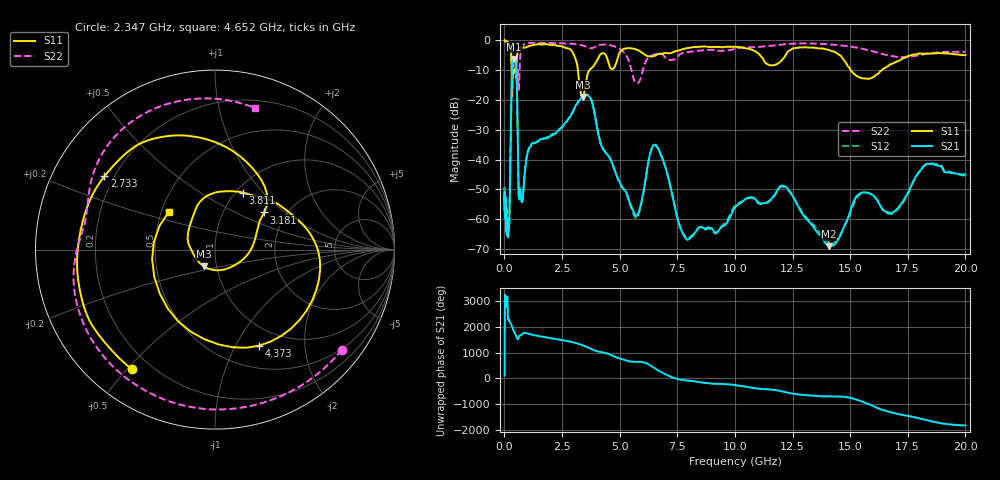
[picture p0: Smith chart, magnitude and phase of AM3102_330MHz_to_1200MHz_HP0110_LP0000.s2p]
! Date/Time: Tue, Sep 11, 2018 5:14 PM
! Network Analyzer: Agilent Technologies E8362B Rev: A.07.50.63
! Sweep from 0.010 to 20.000 GHz, 1601 Points, Sweep Type: LOG
! Power Supply: 4.949 V, 0.001 A
# Hz S DB R 50
!freq MagS11 AngS11 MagS21 AngS21 MagS12 AngS12 MagS22 AngS22
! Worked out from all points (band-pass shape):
!   1601 points, 10 MHz to 20 GHz, reference 50 ohm
!   highest |S21| = -6.20 dB at 420.4 MHz (marker M1); lowest = -69.0 dB at 14.07 GHz (marker M2)
!   |S21| within 3 dB of the highest: 339.9 MHz to 516.9 MHz (177 MHz wide, 41.3 % of centre)
!   lowest |S11| = -19.0 dB at 3.4 GHz (marker M3), VSWR 1.25, Z = 43.4 - j8.18 ohm
!   |S11| at or under -10 dB: 315.1 MHz to 377.6 MHz (62.48 MHz wide, 18 % of centre); 3.19 GHz to 3.687 GHz (496.7 MHz wide, 14.4 % of centre); 15.03 GHz to 16.37 GHz (1.34 GHz wide, 8.54 % of centre)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
!   |S22| runs from -16.5 to -0.2 dB; largest |S21 - S12| = 0.0059
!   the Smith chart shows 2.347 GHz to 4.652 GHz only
!   S11 on the Smith chart (normalised r, x): 2.347 GHz: 0.13, -0.52; 2.733 GHz: 0.16, +0.29; 3.181 GHz: 1.55, +0.73; 3.811 GHz: 1.07, +0.78; 4.373 GHz: 0.76, -1.25; 4.652 GHz: 0.55, +0.26
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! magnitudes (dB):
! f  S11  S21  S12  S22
! 10 MHz  0.0  -53.3  -50.3  -0.2
! 35.55 MHz  0.0  -58.5  -56.7  -0.3
! 126.4 MHz  -0.4  -65.4  -63.1  -0.7
! 217.2 MHz  -1.4  -58.5  -59.9  -1.5
! 420.4 MHz  -10.9  -6.2  -6.2  -7.1
! 447.2 MHz  -10.1  -6.3  -6.4  -7.2
! 530.6 MHz  -7.5  -11.7  -11.7  -12.5
! 635.6 MHz  -2.4  -53.2  -53.5  -15.9
! 1.59 GHz  -1.4  -33.1  -33.1  -0.8
! 2.347 GHz  -1.8  -30.0  -30.4  -0.9
! 2.733 GHz  -2.6  -26.8  -27.0  -1.0
! 3.181 GHz  -9.3  -20.7  -20.9  -1.3
! 3.4 GHz  -19.0  -18.7  -18.9  -1.7
! 3.811 GHz  -9.0  -20.9  -20.8  -2.6
! 4.373 GHz  -4.6  -37.4  -37.4  -1.4
! 4.652 GHz  -9.6  -40.7  -40.7  -1.7
! 5.652 GHz  -2.9  -58.3  -59.1  -13.7
! 6.549 GHz  -5.1  -35.0  -35.2  -4.6
! 7.882 GHz  -2.7  -66.6  -66.3  -4.0
! 12.09 GHz  -6.1  -48.7  -49.0  -1.3
! 14.07 GHz  -3.2  -69.0  -67.7  -1.3
! 20 GHz  -4.9  -45.0  -45.5  -3.8
